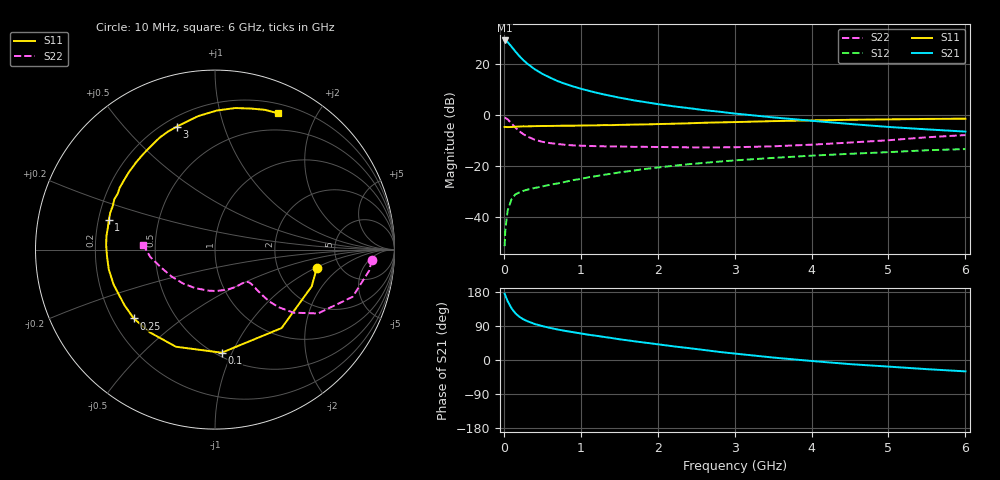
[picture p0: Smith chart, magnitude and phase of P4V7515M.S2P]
! SIEMENS Small Signal Semiconductors
! BFP182
! Si NPN RF Bipolar Junction Transistor in SOT143
! VCE = 0.75 V  IC = 15 mA
! Common Emitter S-Parameters:  March  1996
# GHz  S  MA  R  50
!  f  S11  S21  S12  S22
! GHz  MAG  ANG  MAG  ANG  MAG  ANG  MAG  ANG
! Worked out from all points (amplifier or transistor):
!   36 points, 10 MHz to 6 GHz, reference 50 ohm
!   highest |S21| = 29.0 dB at 10 MHz (marker M1)
!   |S21| within 3 dB of that: start of sweep to 115.3 MHz
!   unconditionally stable (mu >= 1): start of sweep to 10.63 MHz; 424.1 MHz to end of sweep
!   at 250 MHz: K = 0.67, MSG = 25.6 dB, |S12| = -29.8 dB
!   at 1.4 GHz: K = 1.69, MAG = 10.3 dB, |S12| = -23.1 dB
!   at 6 GHz: K = 1.36, MAG = -0.2 dB, |S12| = -13.4 dB
!   S11 on the Smith chart (normalised r, x): 10 MHz: 3.36, -1.05; 100 MHz: 0.53, -0.91; 250 MHz: 0.29, -0.34; 1 GHz: 0.24, +0.13; 3 GHz: 0.25, +0.71; 6 GHz: 0.30, +1.52
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0.01  0.5759 -10.5  28.24 174.9  0.0027 80.6  0.8752 -3.8
0.02  0.5765 -20.8  28.2 170.0  0.0058 80.4  0.8669 -7.8
0.05  0.5734 -49.7  26.3 155.1  0.0135 69.7  0.811 -18.9
0.1  0.5756 -86.3  21.36 136.5  0.0223 53.7  0.6751 -31.8
0.15  0.5833 -111.9  17.22 123.3  0.0278 46.8  0.5608 -38.8
0.2  0.5866 -128.0  14.09 114.3  0.0303 42.1  0.4771 -42.2
0.25  0.5932 -139.7  11.8 107.8  0.0324 39.8  0.4203 -43.6
0.3  0.592 -148.3  10.09 102.9  0.0342 39.3  0.3787 -43.9
0.4  0.5977 -161.0  7.768 95.1  0.037 39.8  0.3252 -43.8
0.5  0.6021 -169.5  6.29 89.5  0.0396 39.7  0.2952 -43.4
0.6  0.6028 -176.4  5.314 84.7  0.0428 40.8  0.279 -43.4
0.7  0.6071 177.6  4.531 80.5  0.0455 42.8  0.2674 -43.7
0.8  0.6096 172.8  3.999 76.7  0.0488 44.0  0.2586 -44.4
1  0.6148 164.2  3.223 70.1  0.0556 45.6  0.2483 -46.6
1.1  0.6186 160.6  2.946 66.7  0.0598 46.2  0.2453 -48.2
1.5  0.633 147.1  2.156 54.8  0.0745 46.8  0.2396 -55.6
2.2  0.6665 126.6  1.464 36.2  0.1004 43.5  0.2326 -73.6
3  0.7175 107.3  1.056 17.0  0.1279 37.2  0.2315 -99.2
3.5  0.7496 97.2  0.887 6.5  0.1433 32.6  0.2414 -117.0
4.5  0.7966 81.9  0.659 -10.9  0.1722 23.7  0.286 -148.9
5.5  0.8271 70.3  0.517 -24.2  0.2022 14.9  0.3622 -173.3
6  0.8365 65.1  0.468 -30.0  0.2132 9.6  0.4002 176.2
